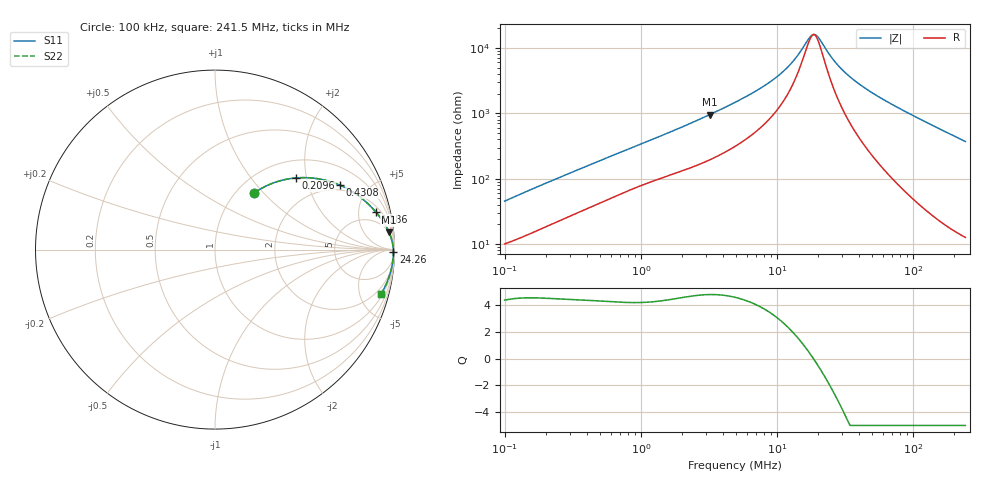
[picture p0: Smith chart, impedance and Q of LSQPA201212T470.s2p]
! LSQPA201212T470  S-PARAMETER MODEL  ( General Type )
! Model Generated by TAIYO YUDEN Corporation (http://www.ty-top.com)
! Version 2.0
! TAIYO YUDEN Control No. 100810NF17SB-FAC
! Copyright(c) 2007 TAIYO YUDEN CO.,LTD. All Rights Reserved.
! Product Description (link to TY-COMPAS)
! https://ds.yuden.co.jp/TYCOMPAS/or/detail?pn=LSQPA201212T470K&u=M
! Products Name : Inductors
! Characteristics :
!  Inductance : 47 uH , SRF(min) : 11 MHz , DC Resistance(max) : 7.54 Ohm
!  Rated Current : Saturation :120 mA , Temp Rise : 150 mA (40 degC)
!  Case Size : 2.0 x 1.25 / 0.079 x 0.049 [mm/inch] , Thickness : 1.25 / 0.049 [mm/inch]
!  (Conditions: Temperature = 25 degC , DC Bias Current/Voltage = 0A / 0V)
! External Node Assignments :
!  1  o---GGG---o  2
! GND o---------o GND
! Frequency Range : 0.1MHz  -  241.513628MHz  [ 402 STEP ]
# MHz S RI R 50
! Freq[MHz].  S11 Real  S11 Imag  S21 Real  S21 Imag  S12 Real  S12 Imag  S22 Real  S22 Imag
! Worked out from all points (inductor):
!   401 points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, 100 kHz to 241.5 MHz, reference 50 ohm
!   read as one part in series: L = 69.2 uH near 104 kHz
!   highest Q = 4.81 at 3.202 MHz (marker M1), where L = 46.4 uH
!   self-resonance near 18.47 MHz
!   S11 on the Smith chart (normalised r, x): 100 kHz: 1.20, +0.89; 209.6 kHz: 1.38, +1.73; 430.8 kHz: 1.74, +3.23; 1.186 MHz: 2.79, +7.62; 24.26 MHz: open; 241.5 MHz: 1.25, -7.40
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0.1  0.2182 0.3147  0.7818 -0.3147  0.7818 -0.3147  0.2182 0.3147
0.209594  0.4512 0.3993  0.5488 -0.3993  0.5488 -0.3993  0.4512 0.3993
0.368674  0.6474 0.3776  0.3526 -0.3776  0.3526 -0.3776  0.6474 0.3776
0.430826  0.6951 0.3599  0.3049 -0.3599  0.3049 -0.3599  0.6951 0.3599
0.701028  0.814 0.2887  0.186 -0.2887  0.186 -0.2887  0.814 0.2887
1.185998  0.8953 0.2105  0.1047 -0.2105  0.1047 -0.2105  0.8953 0.2105
1.359207  0.9106 0.1921  0.0894 -0.1921  0.0894 -0.1921  0.9106 0.1921
3.201909  0.9693 0.0974  0.0307 -0.0974  0.0307 -0.0974  0.9693 0.0974
4.914404  0.9815 0.0644  0.0185 -0.0644  0.0185 -0.0644  0.9815 0.0644
7.691127  0.9884 0.0383  0.0116 -0.0383  0.0116 -0.0383  0.9884 0.0383
10.7094  0.9914 0.0227  0.00861 -0.0227  0.00861 -0.0227  0.9914 0.0227
13.26771  0.9926 0.0136  0.00736 -0.0136  0.00736 -0.0136  0.9926 0.0136
17.08998  0.9936 0.00328  0.0064 -0.00328  0.0064 -0.00328  0.9936 0.00328
18.11814  0.9938 0.000922  0.00625 -0.000922  0.00625 -0.000922  0.9938 0.000922
18.83772  0.9938 -0.000655  0.00616 0.000655  0.00616 0.000655  0.9938 -0.000655
19.97102  0.9939 -0.00303  0.00605 0.00303  0.00605 0.00303  0.9939 -0.00303
24.26464  0.9941 -0.0111  0.00585 0.0111  0.00585 0.0111  0.9941 -0.0111
28.91279  0.9941 -0.0188  0.00588 0.0188  0.00588 0.0188  0.9941 -0.0188
35.81962  0.9938 -0.029  0.00622 0.029  0.00622 0.029  0.9938 -0.029
66.79689  0.99 -0.0681  0.01 0.0681  0.01 0.0681  0.99 -0.0681
129.5109  0.9743 -0.138  0.0257 0.138  0.0257 0.138  0.9743 -0.138
241.5136  0.9248 -0.2472  0.0752 0.2472  0.0752 0.2472  0.9248 -0.2472
